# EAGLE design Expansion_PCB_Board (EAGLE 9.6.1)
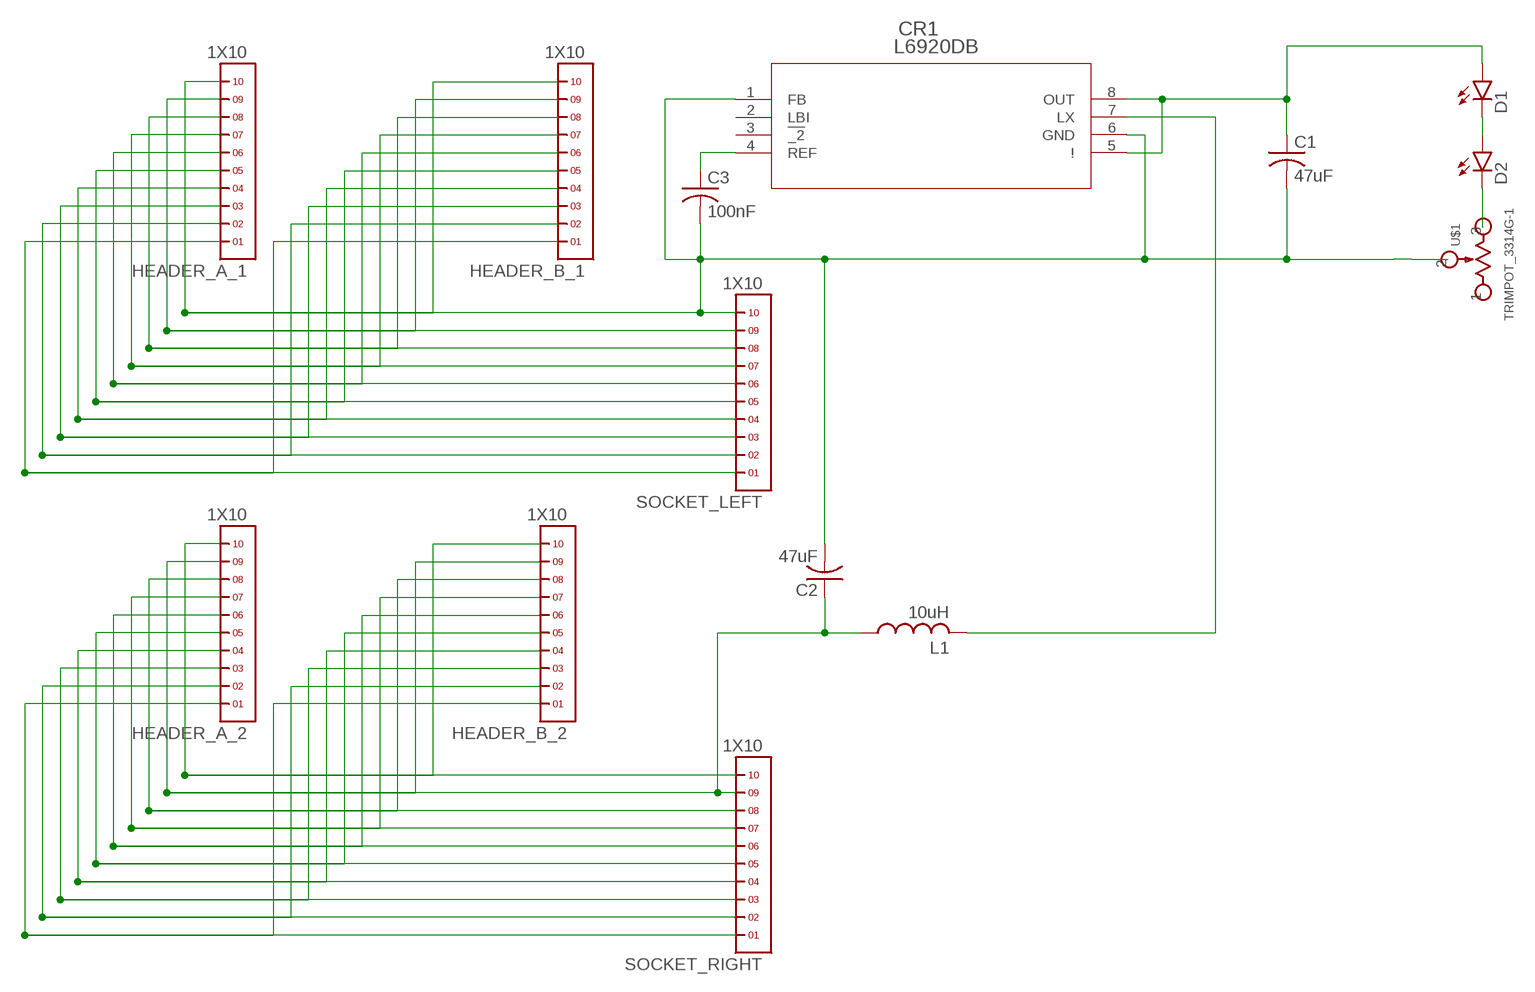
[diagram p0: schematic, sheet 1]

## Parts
C1  47uF  C-US_1206C1206  [C1206]
C2  47uF  C-US_1206C1206  [C1206]
C3  100nF  C-US_1206C1206  [C1206]
CR1  L6920DB  [MSOP-8]
D1  SFH4243-Q1R2  [SFH4243-Q1R2]
D2  SFH4243-Q1R2  [SFH4243-Q1R2]
HEADER_A_1  1X10  [1X10]
HEADER_A_2  1X10  [1X10]
HEADER_B_1  1X10  [1X10]
HEADER_B_2  1X10  [1X10]
L1  10uH  L-US_1210R1210  [R1210]
SOCKET_LEFT  1X10  [1X10]
SOCKET_RIGHT  1X10  [1X10]
U$1  TRIMPOT_3314G-1  [3314G-1]

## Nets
N$1: HEADER_A_1.1 HEADER_B_1.1 SOCKET_LEFT.1
N$2: HEADER_A_1.2 HEADER_B_1.2 SOCKET_LEFT.2
N$3: HEADER_A_1.3 HEADER_B_1.3 SOCKET_LEFT.3
N$4: HEADER_A_1.5 HEADER_B_1.5 SOCKET_LEFT.5
N$5: HEADER_A_1.4 HEADER_B_1.4 SOCKET_LEFT.4
N$6: HEADER_A_2.1 HEADER_B_2.1 SOCKET_RIGHT.1
N$7: HEADER_A_1.6 HEADER_B_1.6 SOCKET_LEFT.6
N$8: HEADER_A_2.2 HEADER_B_2.2 SOCKET_RIGHT.2
N$9: HEADER_A_2.3 HEADER_B_2.3 SOCKET_RIGHT.3
N$10: HEADER_A_1.7 HEADER_B_1.7 SOCKET_LEFT.7
N$11: HEADER_A_2.4 HEADER_B_2.4 SOCKET_RIGHT.4
N$12: HEADER_A_2.5 HEADER_B_2.5 SOCKET_RIGHT.5
N$13: HEADER_A_1.8 HEADER_B_1.8 SOCKET_LEFT.8
N$14: HEADER_A_2.6 HEADER_B_2.6 SOCKET_RIGHT.6
N$15: HEADER_A_2.7 HEADER_B_2.7 SOCKET_RIGHT.7
N$16: HEADER_A_1.9 HEADER_B_1.9 SOCKET_LEFT.9
N$17: HEADER_A_2.8 HEADER_B_2.8 SOCKET_RIGHT.8
N$18: C2.1 HEADER_A_2.9 HEADER_B_2.9 L1.1 SOCKET_RIGHT.9
N$19: C1.2 C2.2 C3.2 CR1.1(FB) CR1.6(GND) HEADER_A_1.10 HEADER_B_1.10 SOCKET_LEFT.10 U$1.2
N$20: HEADER_A_2.10 HEADER_B_2.10 SOCKET_RIGHT.10
N$21: C3.1 CR1.4(REF)
N$22: C1.1 CR1.5(!) CR1.8(OUT) D1.A
N$23: CR1.7(LX) L1.2
N$24: D1.K(C) D2.A
N$25: D2.K(C) U$1.3
Unconnected: CR1.2(LBI) CR1.3(!_2) U$1.1

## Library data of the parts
C1-C3 = crazyflie:C-US_1206: CAPACITOR, American symbol
CR1 = crazyflie:L6920DB; BUILT_BY: EMA_UL_Team; MANUFACTURER_PART_NUMBER: L6920DB; VENDOR: STMicroelectronics
D1 D2 = crazyflie:SFH4243-Q1R2: SFH 4243 - High Power Infrared Emitter (940 nm)
HEADER_A_1 HEADER_A_2 HEADER_B_1 HEADER_B_2 SOCKET_LEFT SOCKET_RIGHT = crazyflie:1X10
L1 = crazyflie:L-US_1210: Inductor, American symbol; SPICEPREFIX: L
U$1 = crazyflie:TRIMPOT_3314G-1: Bourns 3314G-1 Trimmer Resistors - SMD https://www.bourns.com/docs/Product-Datasheets/3314.pdf

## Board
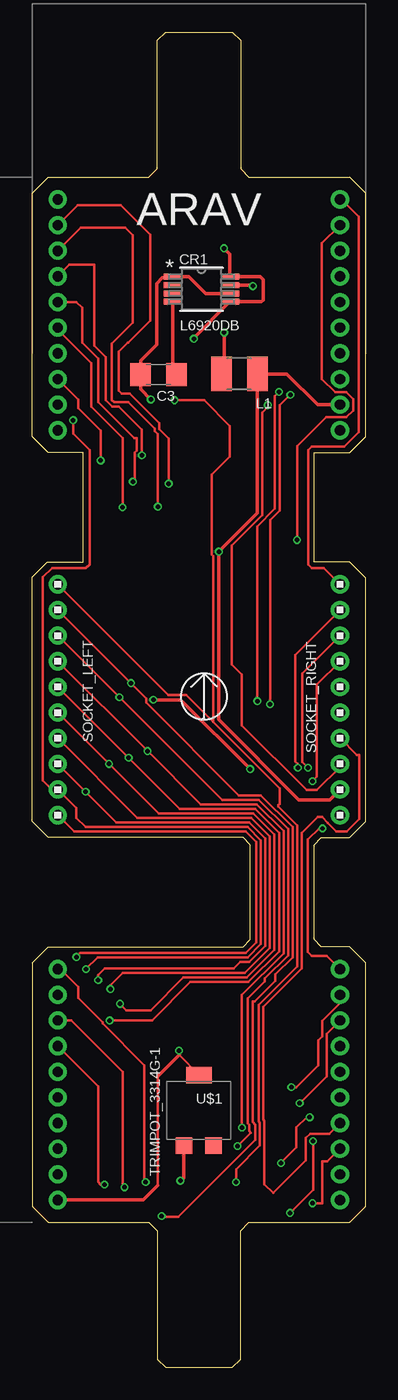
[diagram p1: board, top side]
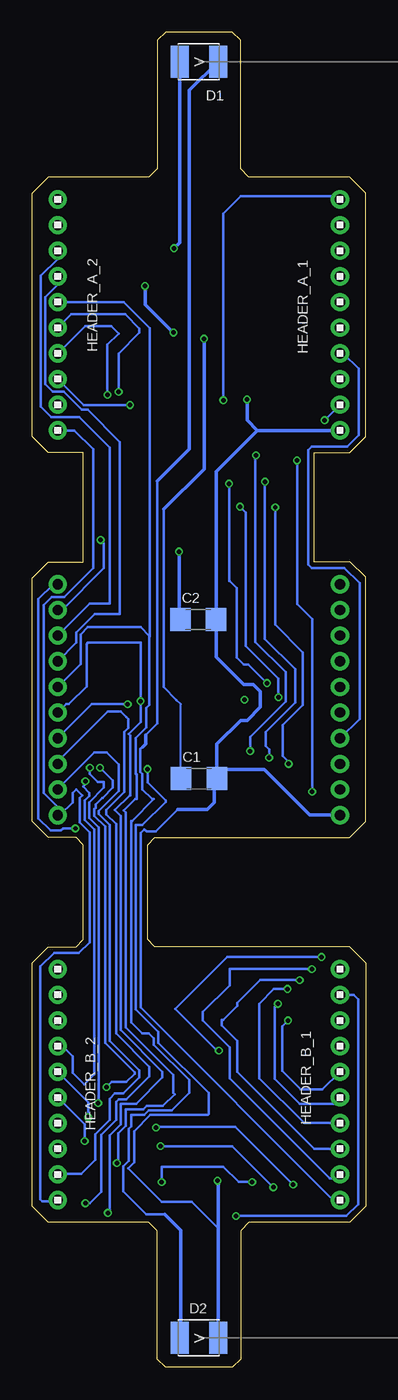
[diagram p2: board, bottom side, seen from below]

Size 26 x 104.1 mm. Coordinates in mm from the lower left corner, seen from the top.
Outline: 0,72.55 0,91.55 1.25,92.8 9.1,92.8 9.75,93.45 9.75,103.45 10.4,104.1 15.6,104.1 16.25,103.45 16.25,93.45 16.9,92.8 24.75,92.8 26,91.55 26,72.55 24.75,71.3 22,71.3 22,62.8 24.75,62.8 26,61.55 26,42.55 24.75,41.3 22.55,41.3 22,40.75 22,33.35 22.55,32.8 24.75,32.8 26,31.55 26,12.55 24.75,11.3 16.9,11.3 16.25,10.65 16.25,0.65 15.6,0 10.4,0 9.75,0.65 9.75,10.65 9.1,11.3 1.25,11.3 0,12.55 0,31.55 1.25,32.8 16.45,32.8 17,33.35 17,40.75 16.45,41.3 1.25,41.3 0,42.55 0,61.6 1.2,62.8 4,62.8 4,71.3 1.25,71.3 0,72.55
Copper layers (1*16): Top 0.035559375mm / dielectric 1.6mm / Bottom 0.035559375mm
Design rules "oshpark-2layer": minimum track width 6mil, minimum drill 10mil, track to track 6mil, track to pad 6mil, pad to pad 6mil, via to via 6mil, smd to smd 6mil, copper to edge 15mil, drill to drill 6mil, minimum pad ring 5mil, minimum via ring 5mil, stop-mask expansion 2.5mil, vias tented up to drill 0mil, thermal gap 10mil

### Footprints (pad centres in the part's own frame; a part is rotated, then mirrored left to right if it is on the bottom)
C1206 = smd 1.6 x 1.8: 1 -1.4,0; 2 1.4,0
MSOP-8 = smd 1.411 x 0.466: 1 -2.223,0.975; 2 -2.223,0.325; 3 -2.223,-0.325; 4 -2.223,-0.975; 5 2.223,-0.975; 6 2.223,-0.325; 7 2.223,0.325; 8 2.223,0.975
SFH4243-Q1R2 = smd 2.5 x 1.4: A 0,1.5; K 0,-1.5
1X10 = drill 0.8 pad 1.422: 1 -9,0; 2 -7,0; 3 -5,0; 4 -3,0; 5 -1,0; 6 1,0; 7 3,0; 8 5,0; 9 7,0; 10 9,0
R1210 = smd 1.6 x 2.7: 1 -1.4,0; 2 1.4,0
3314G-1 = smd 1.3 x 1.3: 1 -1.15,2.75; 3 1.15,2.75 | smd 2 x 1.3: 2 0,-2.75

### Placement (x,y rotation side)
C1  13,45.9 0 bottom
C2  13.05,58.3 0 bottom
C3  9.85,77.4 180 top
CR1  13.2,84.05 0 top
D1  13,101.8 90 bottom
D2  13,2.3 90 bottom
HEADER_A_1  2,82.05 270 bottom
HEADER_A_2  24,82.05 270 bottom
HEADER_B_1  2,22.05 270 bottom
HEADER_B_2  24,22.05 270 bottom
L1  16.15,77.45 180 top
SOCKET_LEFT  2,52.05 270 top
SOCKET_RIGHT  24,52.05 270 top
U$1  13,20.05 180 top

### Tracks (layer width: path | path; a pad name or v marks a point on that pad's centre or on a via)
N$1  (via drill 0.35)
  Top 0.2: v8.85,14.45 8.75,14.55 8.75,23.57 5.5,26.82 5.5,26.9 3.6,28.8 3.6,29.65 2.2,31.05 HEADER_B_1.1 | v15.9,14.45 15.9,15.45 17.75,17.31 17.75,19.08 17.65,19.18 17.65,28.25 20.65,31.25 20.65,42.26 19.2,43.72 19.2,43.85 19.29,43.94 19.29,45.14 14.12,50.32 | SOCKET_LEFT.1 10.62,52.43 12.01,52.43 14.12,50.32 | 14.12,50.32 14.12,63.25 14,63.37 14,69.6 15.4,71 15.4,73.4 13.4,75.4 v11.1,75.4
  Bottom 0.2: v8.85,14.45 9.9,14.45 11.1,15.65 15.9,15.65 v15.9,14.45 | v11.1,75.4 11.1,89.95 9.75,91.3 2.25,91.3 HEADER_A_1.1
N$2  (via drill 0.35)
  Top 0.2: v10.1,11.8 10.15,11.75 11.4,11.75 17.4,17.75 17.4,18.93 17.2,19.13 17.2,28.55 17.35,28.55 18.95,30.15 18.95,30.63 20.3,31.98 20.3,42.12 17.82,44.6 16.12,44.6 8.9,51.82 8.9,52.15 v7.7,53.35 SOCKET_LEFT.2 | v10.65,68.9 10.65,72.4 9.9,73.15 9.9,73.6 7.6,75.9 7,75.9 6.75,76.15 6.75,79.2 7.45,79.9 7.5,79.9 9.2,81.6 9.2,88.3 6.9,90.6 3.55,90.6 HEADER_A_1.2
  Bottom 0.2: v10.1,11.8 1.5,11.8 0.6,12.7 0.6,28.7 0.95,29.05 HEADER_B_1.2 | v7.7,53.35 9.15,54.8 9.5,54.8 10.05,55.35 10.05,60.75 10.6,61.3 10.65,61.3 v10.65,68.9
N$3  (via drill 0.35)
  Top 0.2: v7.2,14.05 7.05,14.2 7.05,23.05 3.05,27.05 HEADER_B_1.3 | v16,17.25 17.05,18.3 16.9,18.45 16.9,18.93 16.8,19.03 16.8,28.75 18.15,30.1 18.15,30.33 19.95,32.13 19.95,41.97 17.67,44.25 14.8,44.25 v6.8,52.25 SOCKET_LEFT.3 | HEADER_A_1.3 3.8,88.85 7.25,88.85 7.85,88.25 7.85,81.45 6.22,79.83 6.22,75.42 6.4,75.25 7.5,75.25 9.55,73.2 9.55,73 9.8,72.75 v9.8,67.1
  Bottom 0.2: v7.2,14.05 10.4,17.25 v16,17.25 | v6.8,52.25 6.8,53.7 9.35,56.25 9.35,66.65 v9.8,67.1
N$4  (via drill 0.35)
  Top 0.2: SOCKET_LEFT.5 v7.53,47.53 11.51,43.54 17.38,43.54 19.24,41.68 19.24,32.42 16.86,30.04 12.34,30.04 9.35,27.05 v6.05,27.05 | HEADER_A_1.5 3.45,83.05 3.9,82.6 3.9,79.9 5.15,78.65 5.15,75.25 7.95,72.45 8.15,72.45 8.15,71.48 8,71.33 8,69.2 v7.85,69.05
  Bottom 0.2: HEADER_B_1.5 3.38,21.68 5.08,21.68 6.5,23.1 6.5,26.6 v6.05,27.05 | v7.53,47.53 7.53,48.17 7.8,48.45 7.8,49.55 5.5,51.85 5.5,54.45 7.85,56.8 v7.85,69.05
N$5  (via drill 0.35)
  Top 0.2: v5.65,14.25 5.35,14.25 5.15,14.45 5.15,21.9 HEADER_B_1.4 | SOCKET_LEFT.4 v9,48.05 13.15,43.89 17.52,43.89 19.59,41.83 19.59,32.28 16.35,29.03 v16.35,18.7 | HEADER_A_1.4 2.9,85.95 4.85,85.95 4.85,79.65 5.75,78.75 5.75,75.4 6.25,74.9 6.75,74.9 8.55,73.1 v8.55,71.1
  Bottom 0.2: v5.65,14.25 10.15,18.75 16.3,18.75 v16.35,18.7 | v9,48.05 9,49.15 6.25,51.9 6.25,52.48 6.25,54.2 8.6,56.55 8.6,71.05 v8.55,71.1
N$6  (via drill 0.35)
  Top 0.2: HEADER_B_2.1 22.95,32.1 21.8,32.1 21.5,32.4 21.5,40.85 21.5,40.88 21.5,41.15 22.37,42.02 v22.63,42.02 | HEADER_A_2.1 24.11,91.05 25.47,89.7 25.47,72.9 24.34,71.78 21.8,71.78 21.52,71.5 21.52,62.6 21.8,62.32 22.73,62.32 SOCKET_RIGHT.1
  Bottom 0.2: v22.63,42.02 23.58,42.02 23.75,41.85 24.55,41.85 25.5,42.8 25.5,59.9 24.35,61.05 SOCKET_RIGHT.1
N$7  (via drill 0.35)
  Top 0.2: v6.85,28.35 7.35,27.85 9.25,27.85 11.79,30.39 16.72,30.39 18.89,32.57 18.89,41.53 17.23,43.19 9.86,43.19 v6,47.05 SOCKET_LEFT.6 | HEADER_A_1.6 2,80.9 4.6,78.3 4.6,74.9 7.05,72.45 v7.05,67.05
  Bottom 0.2: HEADER_B_1.6 2.5,20.55 5.15,20.55 7.1,22.5 7.1,28.1 v6.85,28.35 | v6,47.05 6,47.2 6.45,47.65 6.45,50.1 4.9,51.65 4.9,55.75 7.05,57.9 v7.05,67.05
N$8  (via drill 0.35)
  Top 0.2: HEADER_B_2.2 24,28.41 22.6,27.01 22.6,25.8 22.3,25.5 22.3,23.55 20.6,21.85 v20.2,21.85 | v20.7,46.75 20.7,47.05 20.5,47.26 20.5,55.55 SOCKET_RIGHT.2 | HEADER_A_2.2 22.59,87.64 22.59,77.05 23.62,76.01 24.5,76.01 25.01,75.5 25.01,74.6 24.5,74.09 22.92,74.09 20.65,71.81 v20.65,64.5
  Bottom 0.2: v20.2,21.85 19.8,22.25 18.65,22.25 18,22.9 18,23 20.3,25.3 20.3,42.15 21.15,43 21.15,43.52 21.05,43.62 21.05,43.9 20.55,44.4 20.5,44.4 19.7,45.2 19.7,45.75 v20.7,46.75 | SOCKET_RIGHT.2 23.65,59.05 20.4,62.3 20.4,64.25 v20.65,64.5
N$9  (via drill 0.35)
  Top 0.2: v21.5,46.75 21.05,47.2 21.05,54.1 SOCKET_RIGHT.3 | v20.85,20.6 22.95,22.7 22.95,26 HEADER_B_2.3
  Bottom 0.2: v21.5,46.75 21.5,46.25 20.9,45.65 20.4,45.65 20.4,45.2 21.55,44.05 21.55,42.83 20.8,42.08 20.8,30.55 20.81,30.56 20.81,21.26 20.8,21.25 20.8,20.65 v20.85,20.6 | SOCKET_RIGHT.3 21.5,59.55 19.95,59.55 19.95,71.7 22.34,74.09 24.5,74.09 25.32,74.9 25.32,85.1 24,86.41 HEADER_A_2.3
N$10  (via drill 0.35)
  Top 0.2: SOCKET_LEFT.7 8.21,42.84 17.09,42.84 18.54,41.39 18.54,32.71 16.57,30.75 7.05,30.75 6.1,29.8 v6.1,29.5
  Bottom 0.2: v6.1,29.5 7.15,29.5 8.3,28.35 8.3,22.55 4.8,19.05 HEADER_B_1.7 | HEADER_A_1.7 1.75,79.05 0.55,77.85 0.55,72.68 1.45,71.78 4.2,71.78 4.48,71.5 4.48,62.6 4.2,62.32 1.66,62.32 0.48,61.14 0.48,50.57 SOCKET_LEFT.7
N$11  (via drill 0.35)
  Top 0.2: v21.85,45.7 22.2,46.05 22.2,53.25 SOCKET_RIGHT.4
  Bottom 0.2: HEADER_B_2.4 23.65,25.05 22.85,24.25 22.85,22.95 21.95,22.05 21.17,22.83 21.17,41.95 21.9,42.68 21.9,44.2 21.55,44.55 21.55,44.8 22.02,45.28 21.85,45.45 v21.85,45.7 | SOCKET_RIGHT.4 22.55,56.5 22.55,57.3 21.1,58.75 19.15,58.75 19.15,72.15 21.67,74.67 22.12,74.67 23.54,76.09 24.4,76.09 24.96,76.65 24.96,83.45 24,84.41 HEADER_A_2.4
N$12  (via drill 0.35)
  Top 0.2: v19.4,15.94 20.6,17.14 20.6,18.7 21.4,19.5 v21.63,19.5
  Bottom 0.2: v19.4,15.94 19.36,15.94 19.3,16 19.3,18.25 18.7,18.85 18.7,20.1 17.34,20.1 17.07,20.38 15.82,20.38 14.9,21.3 15,21.4 15,22.8 18.7,26.5 18.7,43.25 18.85,43.4 17.95,44.3 17.85,44.3 17.85,46.22 17.91,46.27 17.91,49.08 17.1,49.89 17.1,51.4 16.85,51.65 16.85,57 | v21.63,19.5 21.63,20.68 HEADER_B_2.5 | 16.85,57 16.82,56.97 16.82,81.02 18.85,83.05 HEADER_A_2.5 | 16.85,57 17.55,57.7 21.65,57.7 22.2,57.15 22.2,54.85 SOCKET_RIGHT.5
N$13  (via drill 0.35)
  Top 0.2: v5.15,30.2 5.15,30.6 5.65,31.1 15.7,31.1 16.21,31.61 16.94,31.61 18.19,32.86 18.19,41.24 16.94,42.49 6.56,42.49 v4.17,44.88 SOCKET_LEFT.8 | HEADER_A_1.8 3.6,75.45 3.6,74.8 5.35,73.05 v5.35,70.7
  Bottom 0.2: HEADER_B_1.8 4,17.05 10,23.05 10,25.45 11.2,26.65 11.2,27.1 11.1,27.1 10,28.2 10,28.4 8.2,30.2 v5.15,30.2 | v4.17,44.88 4.17,58.33 5.35,59.5 v5.35,70.7
N$14  (via drill 0.35)
  Top 0.2: v20.1,12.05 21.9,13.85 v21.9,17.65 | v17.55,51.95 17.55,65.56 18.93,66.94 18.93,75.73 v19.25,76.05
  Bottom 0.2: v20.1,12.05 19.95,12.05 19.95,18.1 19.1,18.95 19.1,20.55 17.9,20.55 15.85,22.6 15.85,23.05 19.1,26.3 19.1,43 19.55,43.45 18.4,44.6 18.35,44.6 18.35,49.25 18.48,49.38 17.55,50.3 v17.55,51.95 17.55,56.5 21.65,56.5 21.75,56.4 21.75,53.1 23.15,51.7 23.35,51.7 SOCKET_RIGHT.6 | v21.9,17.65 21.9,18.95 HEADER_B_2.6 | v19.25,76.05 19.25,79.05 17.65,80.65 17.65,81 18.75,82.1 22.95,82.1 HEADER_A_2.6
N$15  (via drill 0.35)
  Top 0.2: SOCKET_RIGHT.7 25.3,47.75 25.5,47.75 25.5,42.75 24.53,41.78 23.7,41.78 23.05,42.43 23.05,42.45 22.6,42.9 22.25,42.9 21,41.66 21,31.11 18,28.1 18,19.33 18.11,19.22 18.11,14.29 18.8,13.6 21.35,16.15 21.35,17.88 21.67,18.2 23.15,18.2 HEADER_B_2.7 | v18.55,51.7 18.55,66.07 19.28,66.8 19.28,75.03 20.1,75.85 v20.12,75.83
  Bottom 0.2: SOCKET_RIGHT.7 21.35,51.7 v18.55,51.7 | v20.12,75.83 20.12,79.72 19.25,80.6 19.82,81.17 21.88,81.17 HEADER_A_2.7
N$16  (via drill 0.35)
  Top 0.2: v4.2,31.05 5.12,31.97 16.8,31.97 17.83,33 17.83,41.09 16.8,42.13 4.17,42.13 3.45,42.85 3.45,43.6 SOCKET_LEFT.9 1.55,45.05 0.85,45.75 0.85,61.6 1.57,62.32 4.2,62.32 4.48,62.6 4.48,71.5 3.2,72.78 v3.2,73.85
  Bottom 0.2: v4.2,31.05 10.6,31.05 10.6,29.8 12.7,27.7 12.7,27.05 10.6,24.95 10.6,22.55 2.8,14.75 2.3,14.75 HEADER_B_1.9 | HEADER_A_1.9 3.05,74 3.2,74 v3.2,73.85
N$17  (via drill 0.35)
  Top 0.2: v21.85,12.8 22.6,12.8 22.6,16.05 23,16.05 HEADER_B_2.8 | v18.38,75.03 18.45,74.95 17.93,74.43 17.93,66.44 15.55,64.06 15.55,54.8 16.35,54 16.35,50.05 21.4,45 22.2,45 24,46.8 SOCKET_RIGHT.8
  Bottom 0.2: v18.38,75.03 21.98,75.03 HEADER_A_2.8 | v21.85,12.8 21.5,12.8 20.6,13.7 20.6,18.15 19.45,19.3 19.45,20.7 19.25,20.9 18.65,20.9 16.85,22.7 16.85,23.45 19.45,26.05 19.45,42.35 20.23,43.12 20.23,43.45 18.83,44.85 18.83,49.52 18.5,49.85 18.5,50.55 18.68,50.72 19.1,51.15 20.1,51.15 24,47.25 SOCKET_RIGHT.8
N$18  (via drill 0.35)
  Top 0.254: HEADER_A_2.9 22.25,75.05 19.85,77.45 L1.1 17.55,66.6 v14.55,63.6 14.55,50.5 20.8,44.25 23.2,44.25 SOCKET_RIGHT.9
  Bottom 0.2: HEADER_B_2.9 23.95,15.1 22.15,15.1 21.07,16.18 21.07,18.17 19.95,19.3 19.95,20.95 19.55,21.35 18.9,21.35 17.65,22.6 17.65,23.15 19.95,25.45 19.95,42.3 20.8,43.15 20.8,43.38 19.25,44.92 19.25,47 20.2,47.95 21.15,47.95 24,45.1 SOCKET_RIGHT.9
  Bottom 0.254: v14.55,63.6 14.55,58.4 C2.1
N$19  (via drill 0.35)
  Top 0.152: U$1.2 11.45,24.35
  Top 0.2: SOCKET_LEFT.10 3.27,41.78 16.65,41.78 17.48,40.95 17.48,33.15 16.65,32.32 3.77,32.32 v3.45,32 | v11.45,24.7 11.45,24.35 | 9.8,22.7 9.8,14.2
  Top 0.254: HEADER_B_1.10 8.65,13.05 9.8,14.2 | 9.8,22.7 10.93,23.83 11.45,24.35 | CR1.6 13.53,83.72 12.22,85.02 CR1.1 10.89,84.94 10.13,84.94 9.7,84.5 9.7,79.75 8.45,78.5 C3.2 8.45,76.25 v9.25,75.45
  Bottom 0.2: 2.55,13.05 17.55,28.05 17.55,41.65 17.25,41.95 17.08,41.78 16.37,41.78 14.65,43.5 | v3.45,32 10.8,32 14.85,27.95 11.53,24.62 v11.45,24.7
  Bottom 0.254: HEADER_A_1.10 8.45,73.05 | 8.45,73.05 11.65,69.85 C2.2 11.65,55.4 9.5,53.25 8.75,53.25 8.2,52.7 8.2,51.5 9.25,50.45 9.75,50.45 11.6,48.6 C1.2 | C1.2 10.9,46.6 7.9,46.6 4.35,43.05 SOCKET_LEFT.10 | C1.2 11.8,45.7 11.8,44.05 12.35,43.5 14.65,43.5 | 2.55,13.05 HEADER_B_1.10 | v9.25,75.45 9.25,73.85 8.45,73.05
N$20
  Bottom 0.2: HEADER_B_2.10 24.1,12.95 25.2,12.95 25.35,13.1 25.35,31.25 24.28,32.32 22.35,32.32 21.52,33.15 21.52,41.7 22.3,42.48 22.3,44.4 22.1,44.6 22.57,45.08 22.85,44.8 22.85,44.05 23.85,43.05 SOCKET_RIGHT.10 24,43.69 25.1,44.78 25.1,59.42 24.45,60.06 23.49,60.06 21.25,62.3 21.25,71.6 22.7,73.05 HEADER_A_2.10
N$21
  Top 0.254: CR1.4 10.98,77.67 C3.1
N$22  (via drill 0.35)
  Top 0.254: v14.95,87.25 15.42,86.78 CR1.8 17.77,85.02 18,84.8 18,83.2 17.88,83.08 CR1.5 12.6,80.25 v12.6,80.2
  Bottom 0.152: C1.1 14.4,51.7 14.75,52.05
  Bottom 0.2: 15.75,66.9 15.75,53.05 14.75,52.05
  Bottom 0.254: D1.A 14.5,87.7 v14.95,87.25 | v12.6,80.2 12.6,70.05 15.75,66.9
N$23  (via drill 0.35)
  Top 0.254: CR1.7 17.18,84.38 17.2,84.35 v17.2,84.3 | v14.97,80.67 14.97,77.67 L1.2
  Bottom 0.254: v17.2,84.3 17.2,82.85 15,80.65 v14.97,80.67
N$24
  Bottom 0.2: 15.65,11.95 17.1,11.95 18.88,13.73 18.88,15.67 18.45,16.1 18.45,18.6 18.25,18.8 18.25,19.7 17.25,19.7 16.92,20.03 15.12,20.03 13.75,21.4 13.75,22.4 16.5,25.15 16.5,25.65 16.9,26.05 17.41,26.05 18.25,26.9 18.25,42.6 18.2,42.6 16.5,44.3 16.65,44.3 17.4,45.05 17.4,46.27 17.55,46.42 17.55,48.2 17.38,48.38 | 16.25,69.1 16.25,50.2 17.15,49.3
  Bottom 0.254: D1.K 13.75,99.55 13.75,71.6 16.25,69.1 | 15.65,11.95 14.4,10.7 14.4,2.4 D2.A | 17.15,49.3 17.15,48.6 17.38,48.38
N$25  (via drill 0.35)
  Top 0.254: v11.55,14.55 11.8,14.8 11.8,17.25 U$1.3 | v9.45,52.05 11.6,52.05 v17,46.65
  Bottom 0.2: 11.5,10.4 11.5,10.85 13.55,12.9 15.9,12.9 18.52,15.53 18.05,16 18.05,18.39 16.77,19.67 12.33,19.67 12.25,19.75 12.25,21.4 16.15,25.3 16.15,26.15 17.9,27.9 17.9,42.3 17.4,42.3 15.6,44.1 15.6,44.2 17,45.6 v17,46.65
  Bottom 0.254: D2.K 11.5,10.4 11.5,14.5 v11.55,14.55

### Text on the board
tPlace: ARAV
